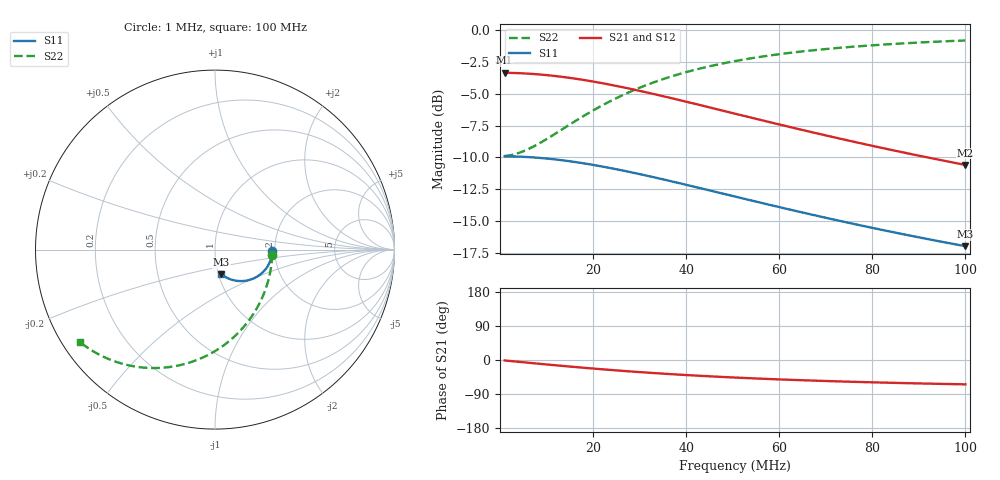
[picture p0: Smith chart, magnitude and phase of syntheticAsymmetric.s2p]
# MHz S RI R 50.0000
! SimSmith 18.3b
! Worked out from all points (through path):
!   100 points, 1 MHz to 100 MHz, reference 50 ohm
!   highest |S21| = -3.35 dB at 1 MHz (marker M1); lowest = -10.6 dB at 100 MHz (marker M2)
!   group delay of S21, straight-line fit = 1.71 ns
!   lowest |S11| = -17.0 dB at 100 MHz (marker M3), VSWR 1.33, Z = 51.6 - j14.5 ohm
!   |S11| at or under -10 dB: 7.22 MHz to end of sweep
!   |S22| runs from -9.9 to -0.8 dB; largest |S21 - S12| = 0
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1  0.3196 -0.00727  0.68 -0.0141  0.68 -0.0141  0.3192 -0.0273
3  0.3184 -0.0217  0.6777 -0.0421  0.6777 -0.0421  0.3146 -0.0818
5  0.316 -0.036  0.673 -0.0698  0.673 -0.0698  0.3057 -0.1353
9  0.3079 -0.0632  0.6574 -0.1227  0.6574 -0.1227  0.2753 -0.2379
11  0.3024 -0.076  0.6466 -0.1475  0.6466 -0.1475  0.2545 -0.2861
14  0.2925 -0.0939  0.6274 -0.1821  0.6274 -0.1821  0.2172 -0.3533
18  0.2769 -0.1149  0.5971 -0.2228  0.5971 -0.2228  0.1584 -0.4323
22  0.2594 -0.1324  0.5631 -0.2568  0.5631 -0.2568  0.0925 -0.4982
26  0.2408 -0.1465  0.5271 -0.2841  0.5271 -0.2841  0.0226 -0.5512
30  0.2219 -0.1573  0.4905 -0.3051  0.4905 -0.3051  -0.0483 -0.5918
34  0.2033 -0.1651  0.4545 -0.3203  0.4545 -0.3203  -0.1183 -0.6215
38  0.1855 -0.1705  0.4198 -0.3307  0.4198 -0.3307  -0.1856 -0.6415
42  0.1685 -0.1737  0.3869 -0.3369  0.3869 -0.3369  -0.2493 -0.6536
46  0.1527 -0.1751  0.3563 -0.3398  0.3563 -0.3398  -0.3088 -0.6591
51  0.1347 -0.1751  0.3212 -0.3396  0.3212 -0.3396  -0.3768 -0.6588
55  0.1215 -0.1738  0.2958 -0.3372  0.2958 -0.3372  -0.4262 -0.6542
59  0.1096 -0.1718  0.2726 -0.3334  0.2726 -0.3334  -0.4712 -0.6467
67  0.0888 -0.1663  0.2322 -0.3226  0.2322 -0.3226  -0.5494 -0.6258
75  0.0717 -0.1595  0.1991 -0.3095  0.1991 -0.3095  -0.6138 -0.6004
84  0.056 -0.1514  0.1687 -0.2938  0.1687 -0.2938  -0.6727 -0.5699
92  0.0447 -0.1442  0.1467 -0.2798  0.1467 -0.2798  -0.7154 -0.5428
100  0.0353 -0.1372  0.1284 -0.2662  0.1284 -0.2662  -0.7509 -0.5164
